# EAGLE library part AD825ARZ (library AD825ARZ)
AD825ARZ, Fast Operational Amplifier 21MHz, 8-Pin SOIC Source: Datasheet
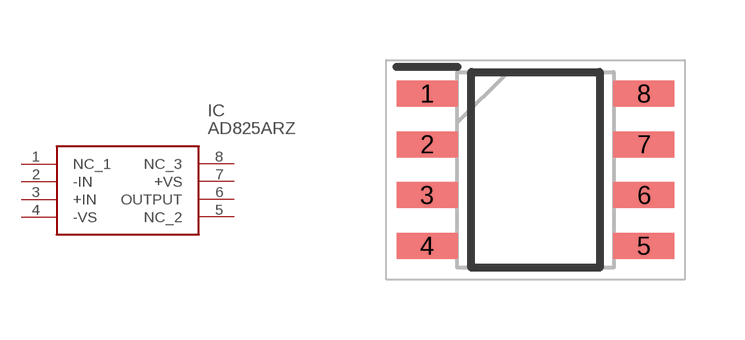
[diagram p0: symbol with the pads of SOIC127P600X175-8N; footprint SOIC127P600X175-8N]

Designator prefix IC

## AD825ARZ (Arrow_Part_Number: AD825ARZ; Arrow_Price-Stock: https://www.arrow.com/en/products/ad825arz/analog-devices?region=nac; Description: AD825ARZ, Fast Operational Amplifier 21MHz, 8-Pin SOIC; Height: 1.75mm; Manufacturer_Name: Analog Devices; Manufacturer_Part_Number: AD825ARZ; Mouser_Part_Number: 584-AD825ARZ; Mouser_Price-Stock: https://www.mouser.co.uk/ProductDetail/Analog-Devices/AD825ARZ?qs=%2FtpEQrCGXCxOEwDf7bhYPw%3D%3D)  [SOIC127P600X175-8N]
1  NC_1
2  -IN
3  +IN
4  -VS
5  NC_2
6  OUTPUT
7  +VS
8  NC_3

## Footprint SOIC127P600X175-8N (pad centres in mm)
. 8-Lead Standard Small Outline Package [SOIC_N]
smd 1.525 x 0.65: 1 -2.712,1.905; 2 -2.712,0.635; 3 -2.712,-0.635; 4 -2.712,-1.905; 5 2.712,-1.905; 6 2.712,-0.635; 7 2.712,0.635; 8 2.712,1.905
